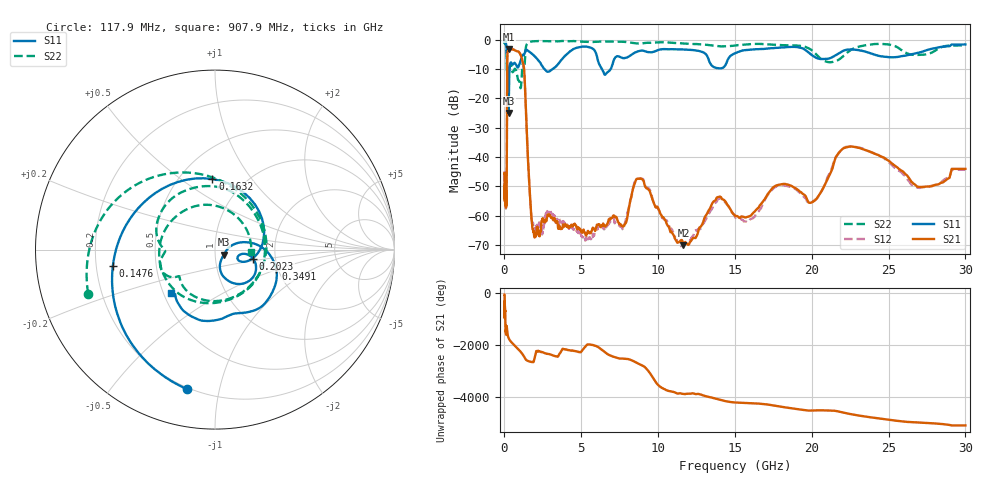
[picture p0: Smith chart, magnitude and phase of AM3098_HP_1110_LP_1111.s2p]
! Date/Time: Thu, Feb 28, 2019 8:47 AM
! Network Analyzer: Agilent Technologies E8364B Rev: A.07.50.67
! Sweep from 0.010 to 30.000 GHz, 1601 Points, Sweep Type: LOG
! Power Supply: 5.023 V, 0.002 A
# Hz S DB R 50
!freq MagS11 AngS11 MagS21 AngS21 MagS12 AngS12 MagS22 AngS22
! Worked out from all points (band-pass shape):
!   1601 points, 10 MHz to 30 GHz, reference 50 ohm
!   highest |S21| = -3.15 dB at 294.5 MHz (marker M1); lowest = -70.0 dB at 11.65 GHz (marker M2)
!   |S21| within 3 dB of the highest: 183.8 MHz to 1.114 GHz (930.4 MHz wide, 143 % of centre)
!   lowest |S11| = -25.0 dB at 265.1 MHz (marker M3), VSWR 1.12, Z = 55 - j3.21 ohm
!   |S11| at or under -10 dB: 169.7 MHz to 330.6 MHz (160.9 MHz wide, 64.3 % of centre); 2.603 GHz to 3.155 GHz (552.1 MHz wide, 19.2 % of centre); 6.348 GHz to 6.915 GHz (567.5 MHz wide, 8.56 % of centre)
!   |S22| runs from -16.6 to -0.5 dB; largest |S21 - S12| = 0.01
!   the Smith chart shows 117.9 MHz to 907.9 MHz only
!   S11 on the Smith chart (normalised r, x): 117.9 MHz: 0.19, -0.80; 147.6 MHz: 0.27, -0.08; 163.2 MHz: 0.71, +0.66; 202.3 MHz: 1.53, -0.16; 349.1 MHz: 1.95, -0.49; 907.9 MHz: 0.55, -0.30
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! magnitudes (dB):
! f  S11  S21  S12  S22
! 10 MHz  -0.4  -45.7  -45.1  -0.6
! 38.04 MHz  -0.3  -51.2  -50.8  -0.9
! 117.9 MHz  -2.0  -56.0  -55.1  -2.5
! 144.7 MHz  -4.3  -51.0  -49.2  -5.3
! 147.6 MHz  -4.8  -48.0  -46.2  -6.1
! 163.2 MHz  -8.1  -20.9  -20.9  -10.9
! 202.3 MHz  -13.2  -4.4  -4.4  -10.9
! 265.1 MHz  -25.0  -3.2  -3.2  -11.1
! 294.5 MHz  -15.4  -3.1  -3.1  -10.5
! 349.1 MHz  -8.9  -3.3  -3.3  -8.8
! 550.5 MHz  -8.4  -3.3  -3.3  -11.0
! 907.9 MHz  -9.3  -4.1  -4.1  -13.9
! 1.27 GHz  -5.3  -9.7  -9.7  -9.9
! 1.74 GHz  -4.6  -59.7  -59.5  -0.7
! 2.084 GHz  -6.3  -65.5  -63.5  -0.5
! 7.926 GHz  -6.2  -62.2  -60.8  -0.8
! 8.848 GHz  -3.8  -47.4  -47.3  -1.3
! 11.65 GHz  -3.3  -70.0  -69.6  -1.3
! 13.88 GHz  -9.7  -53.7  -54.5  -2.2
! 20.1 GHz  -5.6  -55.2  -55.0  -4.1
! 22.56 GHz  -3.3  -36.4  -36.4  -3.5
! 30 GHz  -1.7  -44.1  -44.3  -2.0
